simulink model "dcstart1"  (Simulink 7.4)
settings: Solver=ode45  StartTime=0.0  StopTime=4  MaxStep=.01  RelTol=1e-3
libraries: simulink x1

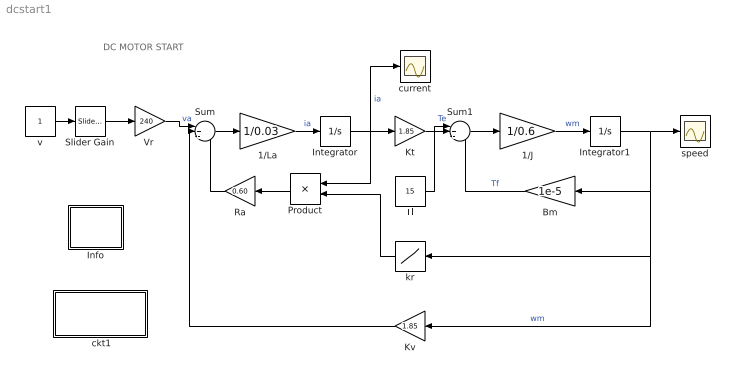
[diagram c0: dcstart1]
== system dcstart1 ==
  note: DC MOTOR START
  " ckt1" : Subsystem
  1/J : Gain  Gain=1/0.6  ParameterDataType=sfix(16)  ParameterScaling=2^0  OutDataType=sfix(16)  OutScaling=2^0
  1/La : Gain  Gain=1/0.03  ParameterDataType=sfix(16)  ParameterScaling=2^0  OutDataType=sfix(16)  OutScaling=2^0
  Bm : Gain  Gain=1e-5  ParameterDataType=sfix(16)  ParameterScaling=2^0  OutDataType=sfix(16)  OutScaling=2^0
  Info : Subsystem
  Integrator : Integrator
  Integrator1 : Integrator
  Kt : Gain  Gain=1.85  ParameterDataType=sfix(16)  ParameterScaling=2^0  OutDataType=sfix(16)  OutScaling=2^0
  Kv : Gain  Gain=1.85  ParameterDataType=sfix(16)  ParameterScaling=2^0  OutDataType=sfix(16)  OutScaling=2^0
  Product : Product  OutDataType=sfix(16)  OutScaling=2^0
  Ra : Gain  Gain=0.60  ParameterDataType=sfix(16)  ParameterScaling=2^0  OutDataType=sfix(16)  OutScaling=2^0
  Slider Gain : simulink/Math Operations/Slider Gain  SystemSampleTime=-1  low=0.5  gain=1  high=1
  Sum : Sum  Inputs=|+--  OutDataType=sfix(16)  OutScaling=2^0
  Sum1 : Sum  Inputs=|+--  OutDataType=sfix(16)  OutScaling=2^0
  Tl : Constant  Value=15  OutDataType=sfix(16)  OutScaling=2^0
  "Vr " : Gain  Gain=240  ParameterDataType=sfix(16)  ParameterScaling=2^0  OutDataType=sfix(16)  OutScaling=2^0
  current : Scope
  kr : Lookup  InputValues=[0 65 65 97.3 97.3 113.5 113.5 121.6 121.6 130]  Table=[12.5 12.5 6.25 6.25 3.125 3.125 1.5625 1.5625 1 1]  OutDataType=sfix(16)  OutScaling=2^0
  speed : Scope
  v : Constant  OutDataType=sfix(16)  OutScaling=2^0
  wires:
  Kv/1 -> Sum/2
  Ra/1 -> Sum/3
  Integrator1/1 -> Bm/1, Kv/1, kr/1, speed/1  "wm"
  Kt/1 -> Sum1/1  "Te"
  Bm/1 -> Sum1/3  "Tf"
  Tl/1 -> Sum1/2
  Product/1 -> Ra/1
  Slider Gain/1 -> "Vr "/1
  "Vr "/1 -> Sum/1  "va"
  v/1 -> Slider Gain/1
  kr/1 -> Product/2
  Integrator/1 -> Kt/1, current/1, Product/1  "ia"
  1/La/1 -> Integrator/1  "ia"
  Sum/1 -> 1/La/1
  Sum1/1 -> 1/J/1
  1/J/1 -> Integrator1/1  "wm"

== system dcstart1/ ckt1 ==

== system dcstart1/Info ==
  note: This demo simulates the starting of a DC motor with automatic starter (5 hp 240V 1200 rpm) rated torque Tr = 30 N.m The starter is simulated by a speed-dependent effective armature resistance using a look-up table.
